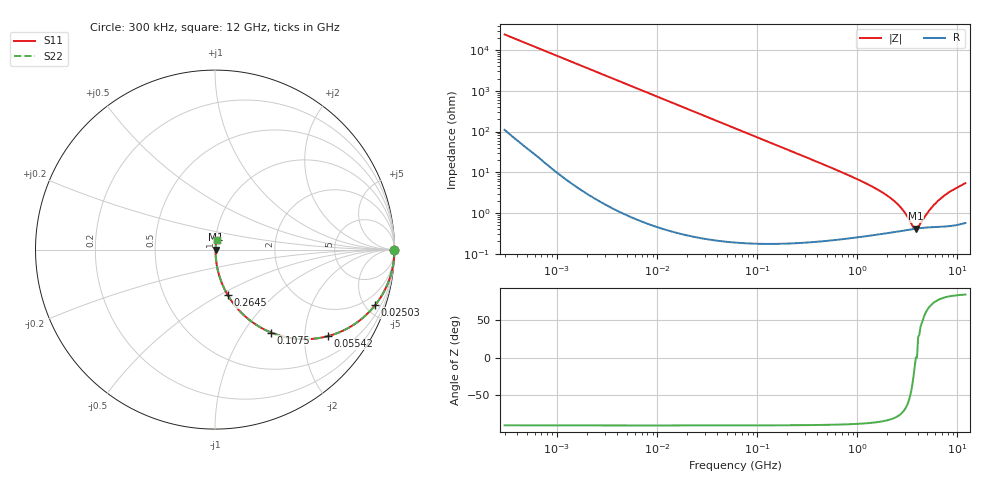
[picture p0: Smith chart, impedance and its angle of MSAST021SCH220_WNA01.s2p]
! MSAST021SCH220_WNA01  S-PARAMETER MODEL  ( General Type )
! Model Generated by TAIYO YUDEN Corporation (http://www.ty-top.com)
! Version 2.0
! TAIYO YUDEN Control No. 181101
! Copyright(c) 2016 TAIYO YUDEN CO.,LTD. All Rights Reserved.
! Product Description (link to TY-COMPAS)
! https://ds.yuden.co.jp/TYCOMPAS/or/detail?pn=MSAST021SCH220JWNA01&u=M
! Products Name : Multilayer Ceramic Capacitors
! Characteristics :
!  Capacitance : 22 pF , Rated Voltage : 25V , TCC : CH / C0H
!  Case Size : 0.25 x 0.125 / 0.0098 x 0.0049 [mm/inch] , Thickness : 0.125 / 0.0049 [mm/inch]
!  (Conditions: Temperature = 25 degC , DC Bias Current/Voltage = 0A / 0V)
! External Node Assignments :
!  1  o---| |---o  2
! GND o---------o GND
! Frequency Range : 0.3MHz  -  12000MHz  [ 401 STEP ]
# MHz S RI R 50
! Freq[MHz].  S11 Real  S11 Imag  S21 Real  S21 Imag  S12 Real  S12 Imag  S22 Real  S22 Imag
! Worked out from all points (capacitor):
!   401 points, 300 kHz to 12 GHz, reference 50 ohm
!   read as one part in series: C = 22 pF near 316.3 kHz
!   lowest |Z| = 412 mohm at 3.841 GHz (marker M1)
!   series resonance near 3.837 GHz, so ESL is about 78 pH
!   S11 on the Smith chart (normalised r, x): 300 kHz: open; 25.03 MHz: 1.01, -5.78; 55.42 MHz: 1.00, -2.61; 107.5 MHz: 1.00, -1.35; 264.5 MHz: 1.00, -0.54; 12 GHz: 1.01, +0.11
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0.3  1 -0.00415  3.61e-05 0.00415  3.61e-05 0.00415  1 -0.00415
1.769972  0.9994 -0.0245  0.00062 0.0245  0.00062 0.0245  0.9994 -0.0245
10.44266  0.9795 -0.1414  0.0205 0.1414  0.0205 0.1414  0.9795 -0.1414
25.03118  0.8929 -0.3089  0.1071 0.3089  0.1071 0.3089  0.8929 -0.3089
37.24419  0.7902 -0.4066  0.2098 0.4066  0.2098 0.4066  0.7902 -0.4066
55.41608  0.6299 -0.4821  0.3701 0.4821  0.3701 0.4821  0.6299 -0.4821
60  0.5922 -0.4906  0.4078 0.4906  0.4078 0.4906  0.5922 -0.4906
107.4644  0.312 -0.462  0.688 0.462  0.688 0.462  0.312 -0.462
164.1901  0.1631 -0.3674  0.8369 0.3674  0.8369 0.3674  0.1631 -0.3674
264.5085  0.0704 -0.2526  0.9296 0.2526  0.9296 0.2526  0.0704 -0.2526
353.9943  0.0411 -0.1939  0.9589 0.1939  0.9589 0.1939  0.0411 -0.1939
1105.905  0.00615 -0.0594  0.9939 0.0594  0.9939 0.0594  0.00615 -0.0594
2088.533  0.00382 -0.0241  0.9962 0.0241  0.9962 0.0241  0.00382 -0.0241
2722.03  0.00376 -0.013  0.9962 0.013  0.9962 0.013  0.00376 -0.013
3026.31  0.00382 -0.00885  0.9962 0.00885  0.9962 0.00885  0.00382 -0.00885
3547.679  0.00399 -0.0028  0.996 0.0028  0.996 0.0028  0.00399 -0.0028
3841.137  0.0041 3.06e-05  0.9959 -3.06e-05  0.9959 -3.06e-05  0.0041 3.06e-05
4050.141  0.00417 0.00218  0.9958 -0.00218  0.9958 -0.00218  0.00417 0.00218
5278.635  0.00455 0.011  0.9955 -0.011  0.9955 -0.011  0.00455 0.011
6524.734  0.00495 0.0202  0.995 -0.0202  0.995 -0.0202  0.00495 0.0202
8281.503  0.00576 0.032  0.9942 -0.032  0.9942 -0.032  0.00576 0.032
12000  0.00846 0.0529  0.9915 -0.0529  0.9915 -0.0529  0.00846 0.0529
